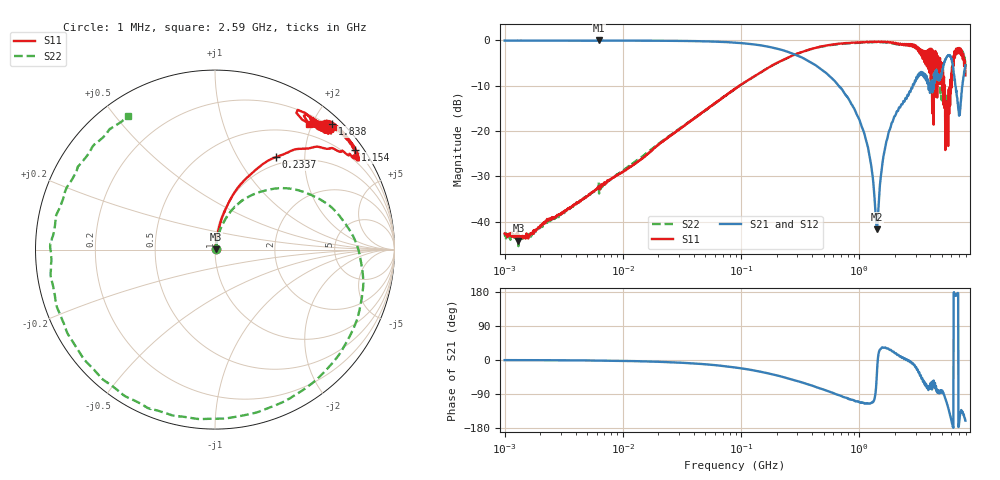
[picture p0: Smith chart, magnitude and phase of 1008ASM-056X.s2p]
!s-Parameter Generated by FASTRON Sdn. Bhd.
!FASTRON P/N : 1008ASM-056X
!Keysight Technologies: E5071C_MY46733604_B.14.02
!Date: Tue Nov 21 11:30:03 2023
!Version  :Rev00  Wed Nov 22 15:48:48 2023
!Data & Calibration Information:
!Freq  S11:SOLT2(ON)  S21:SOLT2(ON)  S12:SOLT2(ON)  S22:SOLT2(ON)
!PortZ  Port1:50+j0  Port2:50+j0
!When reading reference impedance value at option line is always used.
! Remarks : This data is being provided solely for informational purposes.
# Hz S dB R 50
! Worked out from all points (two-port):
!   1599 points, 1 MHz to 7.923 GHz, reference 50 ohm
!   highest |S21| = -0.03 dB at 6.301 MHz (marker M1); lowest = -41.7 dB at 1.411 GHz (marker M2)
!   |S21| within 3 dB of the highest: start of sweep to 278.5 MHz
!   lowest |S11| = -44.2 dB at 1.31 MHz (marker M3), VSWR 1.01, Z = 50.6 + j0.256 ohm
!   |S11| at or under -10 dB: start of sweep to 97.07 MHz; 5.228 GHz to 5.304 GHz (75.39 MHz wide, 1.43 % of centre); 5.305 GHz to 5.909 GHz (604.2 MHz wide, 10.8 % of centre)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
!   |S22| runs from -45.4 to -0.4 dB; largest |S21 - S12| = 0.012
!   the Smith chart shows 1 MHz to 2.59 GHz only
!   S11 on the Smith chart (normalised r, x): 1 MHz: 1.01, +0.00; 233.7 MHz: 0.88, +1.47; 1.154 GHz: 0.22, +3.12; 1.838 GHz: 0.14, +2.29; 2.59 GHz: 0.32, +1.95
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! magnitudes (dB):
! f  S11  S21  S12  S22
! 1 MHz  -42.6  -0.1  -0.1  -42.6
! 1.31 MHz  -44.2  -0.1  -0.1  -45.4
! 4.479 MHz  -35.2  -0.1  -0.1  -35.3
! 6.301 MHz  -32.5  0.0  -0.1  -33.8
! 19.95 MHz  -23.0  -0.1  -0.1  -22.9
! 89.01 MHz  -10.7  -0.5  -0.5  -10.7
! 233.7 MHz  -4.2  -2.3  -2.3  -4.2
! 398.5 MHz  -1.9  -5.0  -5.0  -1.9
! 792.9 MHz  -0.6  -12.5  -12.5  -0.7
! 1.154 GHz  -0.4  -22.4  -22.4  -0.5
! 1.411 GHz  -0.4  -41.7  -41.8  -0.4
! 1.605 GHz  -0.4  -25.6  -25.7  -0.4
! 1.784 GHz  -0.5  -20.1  -20.2  -0.6
! 1.838 GHz  -0.4  -19.3  -19.4  -0.6
! 2.59 GHz  -1.1  -12.1  -12.1  -1.0
! 3.305 GHz  -2.0  -7.6  -7.6  -2.4
! 4.176 GHz  -6.3  -11.0  -11.0  -2.8
! 4.828 GHz  -3.9  -8.7  -8.7  -9.6
! 5.528 GHz  -16.0  -3.6  -3.6  -13.6
! 6.381 GHz  -4.0  -7.9  -7.8  -3.3
! 6.998 GHz  -1.7  -16.6  -16.6  -2.5
! 7.923 GHz  -7.7  -5.5  -5.5  -5.9
